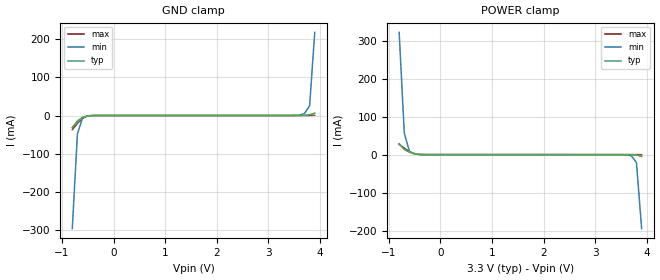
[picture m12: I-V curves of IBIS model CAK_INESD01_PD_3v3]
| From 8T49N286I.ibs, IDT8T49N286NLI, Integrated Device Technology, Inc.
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| 4.00000e+00   -1.39574e-02   -4.76185e-01   -2.49150e-03
| 4.10000e+00   -3.15147e-02   -7.57906e-01   -1.14779e-02
| 4.20000e+00   -2.28020e-01   -1.04025e+00   -2.65085e-02
| 4.30000e+00   -6.05544e-01   -1.32303e+00   -4.22040e-02
| 4.40000e+00   -9.83665e-01   -1.60616e+00   -8.93095e-02
| 4.50000e+00   -1.36232e+00   -1.88960e+00   -5.31450e-01
| 4.60000e+00   -1.74144e+00   -2.17334e+00   -1.01592e+00
| 4.70000e+00   -2.12099e+00   -2.45736e+00   -1.50093e+00
| 4.80000e+00   -2.50093e+00   -2.74165e+00   -1.98638e+00
| 4.90000e+00   -2.88119e+00   -3.02618e+00   -2.47221e+00
| 5.00000e+00   -3.26174e+00   -3.31095e+00   -2.95834e+00
| 5.10000e+00   -3.64255e+00   -3.59594e+00   -3.44470e+00
| 5.20000e+00   -4.02357e+00   -3.88113e+00   -3.93127e+00
| 5.30000e+00   -4.40478e+00   -4.16651e+00   -4.41800e+00
| 5.40000e+00   -4.78614e+00   -4.45206e+00   -4.90488e+00
| 5.50000e+00   -5.16764e+00   -4.73778e+00   -5.39189e+00
| 5.60000e+00   -5.54926e+00   -5.02364e+00   -5.87898e+00
| 5.70000e+00   -5.93098e+00   -5.30964e+00   -6.36615e+00
| 5.80000e+00   -6.31277e+00   -5.59577e+00   -6.85336e+00
| 5.90000e+00   -6.69464e+00   -5.88201e+00   -7.34061e+00
| 6.00000e+00   -7.07656e+00   -6.16836e+00   -7.82788e+00
| 6.10000e+00   -7.45854e+00   -6.45481e+00   -8.31516e+00
| 6.20000e+00   -7.84055e+00   -6.74136e+00   -8.80244e+00
| 6.30000e+00   -8.22259e+00   -7.02799e+00   -9.28972e+00
| 6.40000e+00   -8.60465e+00   -7.31471e+00   -9.77698e+00
| 6.50000e+00   -8.98673e+00   -7.60150e+00   -1.02642e+01
| 6.60000e+00   -9.36883e+00   -7.88836e+00   -1.07515e+01
[Model]   CAK_INESD01_PD_3v3
Model_type   Input
Polarity   Non-Inverting
Vinl = 0.8V
Vinh = 2.0V
|   typ   min   max
C_comp   2pF   1.5pF   2.5pF
|   typ   min   max
[Voltage range]   3.3V   3.135V   3.465V
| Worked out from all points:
|   GND clamp passes 1 mA (typ) near -0.51 V on its own axis
|   POWER clamp passes 1 mA (typ) near -0.44 V on its own axis
[GND_clamp]
|Voltage   I (typ)   I (min)   I (max)
|Note, modeling breaks down at 250mA and above.  This is well beyond the functional   |
|operating range of the device.  Should this scenario occur, catastrophic failure and   |
|possible damage to the device and/or board is of higher concern than the I-V curve   |
|behavior.  The IBIS checker will flag currents in excess of 10A with warnings.  Lines   |
|with currents in excess of 0.35 A have been commented out.  The points still remain|
|available to the user if the user desires to use them.   |
|-3.30000e+00   -9.36883e+00   -7.41795e+00   -1.15553e+01
|-3.20000e+00   -8.98673e+00   -7.13120e+00   -1.10681e+01
|-3.10000e+00   -8.60465e+00   -6.84454e+00   -1.05809e+01
|-3.00000e+00   -8.22259e+00   -6.55796e+00   -1.00937e+01
|-2.90000e+00   -7.84055e+00   -6.27147e+00   -9.60644e+00
|-2.80000e+00   -7.45854e+00   -5.98508e+00   -9.11917e+00
|-2.70000e+00   -7.07656e+00   -5.69880e+00   -8.63189e+00
|-2.60000e+00   -6.69464e+00   -5.41263e+00   -8.14461e+00
|-2.50000e+00   -6.31277e+00   -5.12658e+00   -7.65734e+00
|-2.40000e+00   -5.93098e+00   -4.84067e+00   -7.17007e+00
|-2.30000e+00   -5.54926e+00   -4.55490e+00   -6.68283e+00
|-2.20000e+00   -5.16764e+00   -4.26929e+00   -6.19563e+00
|-2.10000e+00   -4.78614e+00   -3.98385e+00   -5.70849e+00
|-2.00000e+00   -4.40478e+00   -3.69859e+00   -5.22142e+00
|-1.90000e+00   -4.02357e+00   -3.41352e+00   -4.73446e+00
|-1.80000e+00   -3.64255e+00   -3.12867e+00   -4.24763e+00
|-1.70000e+00   -3.26174e+00   -2.84405e+00   -3.76095e+00
|-1.60000e+00   -2.88119e+00   -2.55967e+00   -3.27445e+00
|-1.50000e+00   -2.50093e+00   -2.27556e+00   -2.78816e+00
|-1.40000e+00   -2.12099e+00   -1.99172e+00   -2.30213e+00
|-1.30000e+00   -1.74144e+00   -1.70816e+00   -1.81643e+00
|-1.20000e+00   -1.36232e+00   -1.42492e+00   -1.33112e+00
|-1.10000e+00   -9.83665e-01   -1.14201e+00   -8.46289e-01
|-1.00000e+00   -6.05544e-01   -8.59494e-01   -3.62030e-01
|-9.00000e-01   -2.28020e-01   -5.77510e-01   -5.71068e-02
-800mV    -31.51mA   -296.3mA   -37.05mA
-700mV    -13.96mA   -47.9mA    -20.78mA
-600mV    -4.826mA   -5.935mA   -7.491mA
-500mV    -779.5uA   -884.9uA   -1.121mA
-400mV    -58.36uA   -98.1uA    -62.19uA
3.4V      67.73uA    67.08uA    78.25uA
3.6V      79.25uA    1.239mA    82.85uA
3.7V      274.3uA    5.013mA    85.36uA
3.8V      1.921mA    25.27mA    105.6uA
3.9V      6.27mA     217.7mA    653.2uA
| 4.00000e+00   1.35090e-02   5.06610e-01   3.93491e-03
| 4.10000e+00   2.86495e-02   7.94972e-01   1.06964e-02
| 4.20000e+00   2.42185e-01   1.08363e+00   2.06408e-02
| 4.30000e+00   6.27220e-01   1.37264e+00   3.03092e-02
| 4.40000e+00   1.01272e+00   1.66203e+00   7.71926e-02
| 4.50000e+00   1.39872e+00   1.95179e+00   5.37535e-01
| 4.60000e+00   1.78522e+00   2.24193e+00   1.03072e+00
| 4.70000e+00   2.17221e+00   2.53243e+00   1.52454e+00
| 4.80000e+00   2.55968e+00   2.82330e+00   2.01896e+00
| 4.90000e+00   2.94760e+00   3.11454e+00   2.51397e+00
| 5.00000e+00   3.33598e+00   3.40615e+00   3.00954e+00
| 5.10000e+00   3.72481e+00   3.69812e+00   3.50565e+00
| 5.20000e+00   4.11406e+00   3.99047e+00   4.00228e+00
| 5.30000e+00   4.50374e+00   4.28319e+00   4.49940e+00
| 5.40000e+00   4.89384e+00   4.57629e+00   4.99701e+00
| 5.50000e+00   5.28436e+00   4.86978e+00   5.49507e+00
| 5.60000e+00   5.67529e+00   5.16367e+00   5.99359e+00
| 5.70000e+00   6.06664e+00   5.45797e+00   6.49254e+00
| 5.80000e+00   6.45841e+00   5.75269e+00   6.99193e+00
| 5.90000e+00   6.85059e+00   6.04785e+00   7.49174e+00
| 6.00000e+00   7.24321e+00   6.34345e+00   7.99197e+00
| 6.10000e+00   7.63627e+00   6.63953e+00   8.49262e+00
| 6.20000e+00   8.02978e+00   6.93610e+00   8.99370e+00
| 6.30000e+00   8.42375e+00   7.23318e+00   9.49520e+00
| 6.40000e+00   8.81821e+00   7.53080e+00   9.99715e+00
| 6.50000e+00   9.21316e+00   7.82898e+00   1.04995e+01
| 6.60000e+00   9.60863e+00   8.12774e+00   1.10024e+01
[Power_clamp]
|Voltage   I (typ)   I (min)   I (max)
|Note, modeling breaks down at 250mA and above.  This is well beyond the functional   |
|operating range of the device.  Should this scenario occur, catastrophic failure and   |
|possible damage to the device and/or board is of higher concern than the I-V curve   |
|behavior.  The IBIS checker will flag currents in excess of 10A with warnings.  Lines   |
|with currents in excess of 0.35 A have been commented out.  The points still remain|
|available to the user if the user desires to use them.   |
|-3.30000e+00   9.60863e+00   7.63808e+00   1.18332e+01
|-3.20000e+00   9.21316e+00   7.34026e+00   1.13295e+01
|-3.10000e+00   8.81821e+00   7.04299e+00   1.08263e+01
|-3.00000e+00   8.42375e+00   6.74624e+00   1.03236e+01
|-2.90000e+00   8.02978e+00   6.44999e+00   9.82142e+00
|-2.80000e+00   7.63627e+00   6.15421e+00   9.31963e+00
|-2.70000e+00   7.24321e+00   5.85890e+00   8.81827e+00
|-2.60000e+00   6.85059e+00   5.56402e+00   8.31734e+00
|-2.50000e+00   6.45841e+00   5.26957e+00   7.81684e+00
|-2.40000e+00   6.06664e+00   4.97554e+00   7.31675e+00
|-2.30000e+00   5.67529e+00   4.68190e+00   6.81709e+00
|-2.20000e+00   5.28436e+00   4.38866e+00   6.31786e+00
|-2.10000e+00   4.89384e+00   4.09580e+00   5.81906e+00
|-2.00000e+00   4.50374e+00   3.80332e+00   5.32070e+00
|-1.90000e+00   4.11406e+00   3.51122e+00   4.82279e+00
|-1.80000e+00   3.72481e+00   3.21948e+00   4.32535e+00
|-1.70000e+00   3.33598e+00   2.92811e+00   3.82840e+00
|-1.60000e+00   2.94760e+00   2.63710e+00   3.33195e+00
|-1.50000e+00   2.55968e+00   2.34647e+00   2.83603e+00
|-1.40000e+00   2.17221e+00   2.05620e+00   2.34065e+00
|-1.30000e+00   1.78522e+00   1.76630e+00   1.84584e+00
|-1.20000e+00   1.39872e+00   1.47678e+00   1.35163e+00
|-1.10000e+00   1.01272e+00   1.18763e+00   8.58035e-01
|-1.00000e+00   6.27220e-01   8.98848e-01   3.65067e-01
|-9.00000e-01   2.42185e-01   6.10400e-01   4.21780e-02
-800mV    28.65mA    321.9mA    27.22mA
-700mV    13.51mA    56.43mA    16.88mA
-600mV    6.27mA     8.252mA    7.941mA
-500mV    1.921mA    2.134mA    2.384mA
-300mV    79.25uA    83.14uA    91.24uA
3.5V      -4.022uA   -43.47uA   -806.9nA
3.7V      -58.35uA   -3.051mA   -5.449uA
3.8V      -779.5uA   -21.2mA    -11.73uA
3.9V      -4.826mA   -194.9mA   -182.9uA
